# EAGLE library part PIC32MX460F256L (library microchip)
PIC32MX460F256L edit this description Auto generated by make-symbol-device-package-bsdl.ulp Rev. 25 Source: PIC32MX460F256L.bsdl
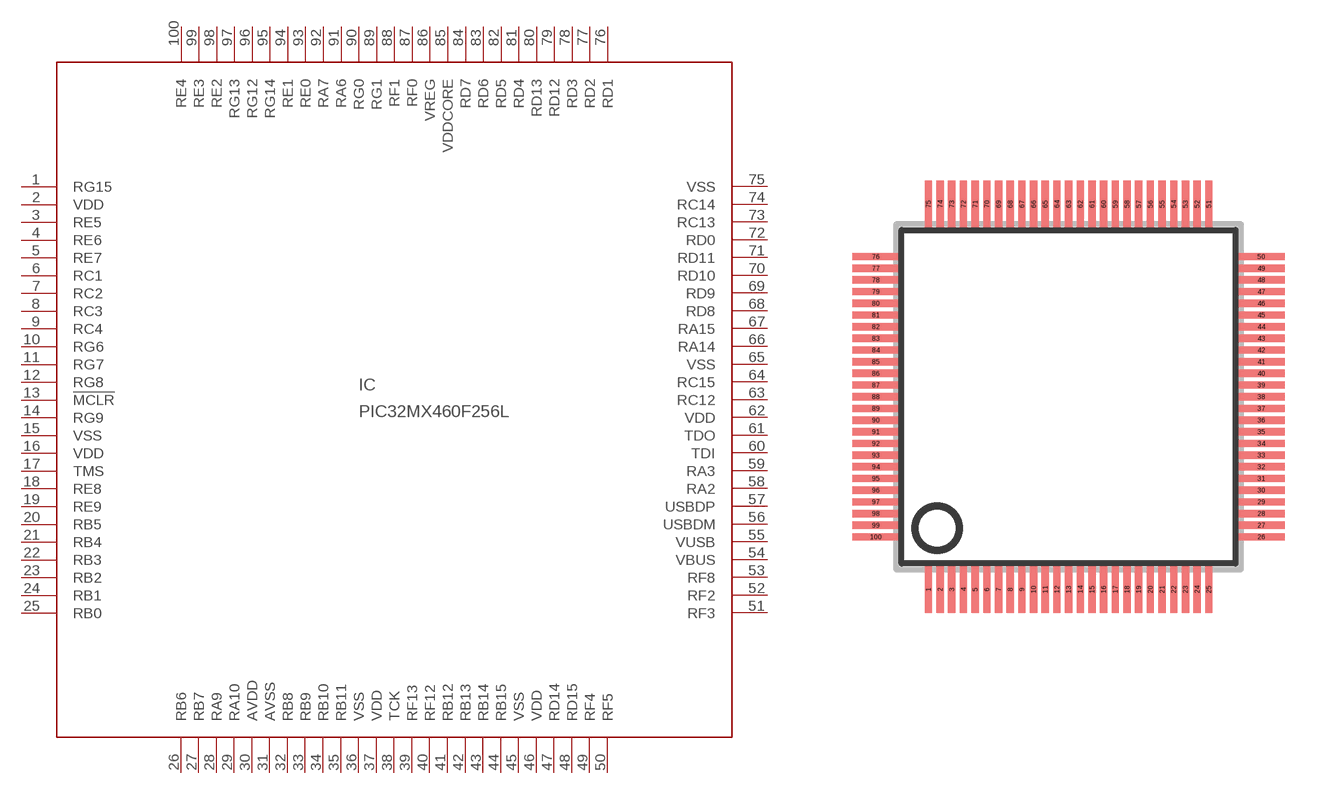
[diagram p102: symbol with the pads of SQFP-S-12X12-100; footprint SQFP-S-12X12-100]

Designator prefix IC

## PIC32MX460F256L (MPN: PIC32MX460F256L-80I/PT; OC_FARNELL: 1778952; OC_NEWARK: 98M1937)  [SQFP-S-12X12-100]
1  RG15
2  VDD  pwr
3  RE5
4  RE6
5  RE7
6  RC1
7  RC2
8  RC3
9  RC4
10  RG6
11  RG7
12  RG8
13  !MCLR  in
14  RG9
15  VSS  pwr
16  VDD  pwr
17  TMS  in
18  RE8
19  RE9
20  RB5
21  RB4
22  RB3
23  RB2
24  RB1
25  RB0
26  RB6
27  RB7
28  RA9
29  RA10
30  AVDD  pwr
31  AVSS  pwr
32  RB8
33  RB9
34  RB10
35  RB11
36  VSS  pwr
37  VDD  pwr
38  TCK  in
39  RF13
40  RF12
41  RB12
42  RB13
43  RB14
44  RB15
45  VSS  pwr
46  VDD  pwr
47  RD14
48  RD15
49  RF4
50  RF5
51  RF3
52  RF2
53  RF8
54  VBUS
55  VUSB  pas
56  USBDM
57  USBDP
58  RA2
59  RA3
60  TDI  in
61  TDO  out
62  VDD  pwr
63  RC12
64  RC15
65  VSS  pwr
66  RA14
67  RA15
68  RD8
69  RD9
70  RD10
71  RD11
72  RD0
73  RC13
74  RC14
75  VSS  pwr
76  RD1
77  RD2
78  RD3
79  RD12
80  RD13
81  RD4
82  RD5
83  RD6
84  RD7
85  VDDCORE  pwr
86  VREG  pas
87  RF0
88  RF1
89  RG1
90  RG0
91  RA6
92  RA7
93  RE0
94  RE1
95  RG14
96  RG12
97  RG13
98  RE2
99  RE3
100  RE4

## Footprint SQFP-S-12X12-100 (pad centres in mm)
QFP100 shrink quad flat pack, square
smd 0.25 x 1.6: 1 -4.8,-6.6; 2 -4.4,-6.6; 3 -4,-6.6; 4 -3.6,-6.6; 5 -3.2,-6.6; 6 -2.8,-6.6; 7 -2.4,-6.6; 8 -2,-6.6; 9 -1.6,-6.6; 10 -1.2,-6.6; 11 -0.8,-6.6; 12 -0.4,-6.6; 13 0,-6.6; 14 0.4,-6.6; 15 0.8,-6.6; 16 1.2,-6.6; 17 1.6,-6.6; 18 2,-6.6; 19 2.4,-6.6; 20 2.8,-6.6; 21 3.2,-6.6; 22 3.6,-6.6; 23 4,-6.6; 24 4.4,-6.6; 25 4.8,-6.6; 51 4.8,6.6; 52 4.4,6.6; 53 4,6.6; 54 3.6,6.6; 55 3.2,6.6; 56 2.8,6.6; 57 2.4,6.6; 58 2,6.6; 59 1.6,6.6; 60 1.2,6.6; 61 0.8,6.6; 62 0.4,6.6; 63 0,6.6; 64 -0.4,6.6; 65 -0.8,6.6; 66 -1.2,6.6; 67 -1.6,6.6; 68 -2,6.6; 69 -2.4,6.6; 70 -2.8,6.6; 71 -3.2,6.6; 72 -3.6,6.6; 73 -4,6.6; 74 -4.4,6.6; 75 -4.8,6.6
smd 1.6 x 0.25: 26 6.6,-4.8; 27 6.6,-4.4; 28 6.6,-4; 29 6.6,-3.6; 30 6.6,-3.2; 31 6.6,-2.8; 32 6.6,-2.4; 33 6.6,-2; 34 6.6,-1.6; 35 6.6,-1.2; 36 6.6,-0.8; 37 6.6,-0.4; 38 6.6,0; 39 6.6,0.4; 40 6.6,0.8; 41 6.6,1.2; 42 6.6,1.6; 43 6.6,2; 44 6.6,2.4; 45 6.6,2.8; 46 6.6,3.2; 47 6.6,3.6; 48 6.6,4; 49 6.6,4.4; 50 6.6,4.8; 76 -6.6,4.8; 77 -6.6,4.4; 78 -6.6,4; 79 -6.6,3.6; 80 -6.6,3.2; 81 -6.6,2.8; 82 -6.6,2.4; 83 -6.6,2; 84 -6.6,1.6; 85 -6.6,1.2; 86 -6.6,0.8; 87 -6.6,0.4; 88 -6.6,0; 89 -6.6,-0.4; 90 -6.6,-0.8; 91 -6.6,-1.2; 92 -6.6,-1.6; 93 -6.6,-2; 94 -6.6,-2.4; 95 -6.6,-2.8; 96 -6.6,-3.2; 97 -6.6,-3.6; 98 -6.6,-4; 99 -6.6,-4.4; 100 -6.6,-4.8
